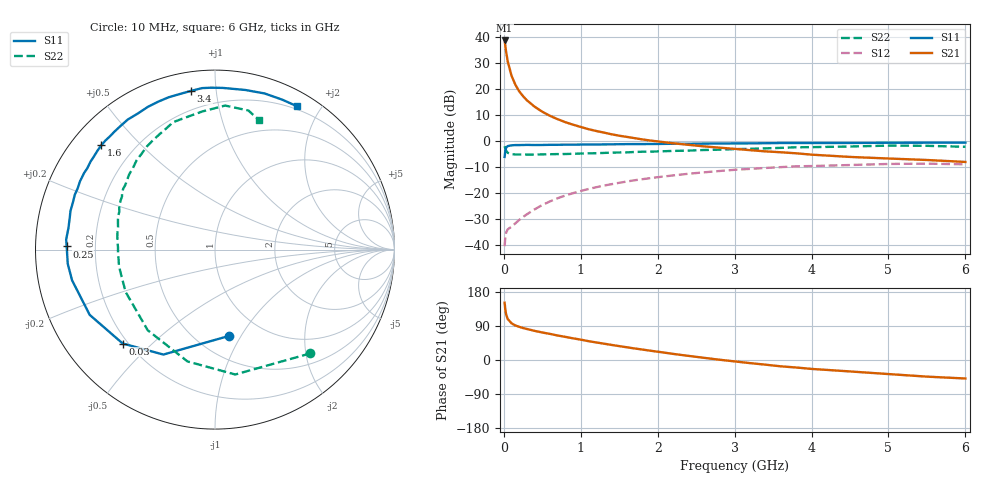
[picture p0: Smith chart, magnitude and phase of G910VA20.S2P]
! SIEMENS Small Signal Semiconductors
! BFG235
! Si NPN RF Bipolar Junction Transistor in SOT223
! VCE = 10 V  IC = 200 mA
! Common Emitter S-Parameters:  July  1994
# GHz  S  MA  R  50
!  f  S11  S21  S12  S22
! GHz  MAG  ANG  MAG  ANG  MAG  ANG  MAG  ANG
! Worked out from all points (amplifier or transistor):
!   40 points, 10 MHz to 6 GHz, reference 50 ohm
!   highest |S21| = 38.6 dB at 10 MHz (marker M1)
!   |S21| within 3 dB of that: start of sweep to 23.6 MHz
!   unconditionally stable (mu >= 1): 410.2 MHz to 1.514 GHz
!   at 200 MHz: K = 0.81, MSG = 24.8 dB, |S12| = -30.5 dB
!   at 1.5 GHz: K = 1.00, MAG = 8.8 dB, |S12| = -16.2 dB
!   at 6 GHz: K = 0.89, MSG = 0.5 dB, |S12| = -9.1 dB
!   S11 on the Smith chart (normalised r, x): 10 MHz: 0.71, -0.89; 30 MHz: 0.18, -0.41; 250 MHz: 0.09, +0.01; 1.6 GHz: 0.09, +0.39; 3.4 GHz: 0.10, +0.86; 6 GHz: 0.16, +1.72
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0.01  0.487 -80.5  85.33 151.2  0.0093 60.6  0.7854 -47.4
0.02  0.6517 -116.2  66.18 132.0  0.0143 47.0  0.705 -80.8
0.03  0.7336 -134.5  51.35 120.4  0.017 40.0  0.6417 -103.8
0.05  0.7872 -152.5  33.88 108.2  0.0196 32.9  0.585 -129.9
0.1  0.8145 -167.9  17.82 96.8  0.0221 36.5  0.5511 -154.6
0.15  0.8242 -174.5  11.94 91.1  0.0256 43.4  0.5415 -164.8
0.2  0.824 -178.1  8.938 87.5  0.0298 48.8  0.5429 -170.3
0.25  0.8266 178.8  7.2 84.3  0.034 52.1  0.5399 -174.0
0.3  0.8311 176.1  6.01 81.8  0.0383 55.4  0.5408 -177.1
0.4  0.8253 171.6  4.522 76.9  0.0476 58.4  0.5405 178.7
0.5  0.828 168.0  3.61 72.6  0.0577 59.8  0.5451 175.4
0.6  0.8335 165.0  3.012 68.9  0.0678 60.2  0.5491 172.3
0.7  0.8345 161.3  2.596 64.6  0.0781 60.2  0.5525 169.5
0.9  0.8377 155.9  2.033 57.2  0.0977 58.1  0.5597 165.0
1.1  0.845 149.6  1.668 49.7  0.1174 55.8  0.5711 160.3
1.6  0.8597 137.4  1.183 33.6  0.1638 47.5  0.5965 150.3
2.2  0.8724 124.0  0.893 16.1  0.2144 36.7  0.6361 138.7
3.2  0.8887 102.8  0.658 -8.2  0.2868 17.5  0.6984 120.2
3.4  0.8943 98.6  0.623 -12.3  0.2983 13.5  0.7124 115.9
4.5  0.9052 79.3  0.487 -30.2  0.3401 -7.2  0.7726 95.3
5.5  0.9155 65.9  0.425 -43.9  0.3614 -25.6  0.797 76.5
6  0.9202 60.1  0.39 -48.8  0.3508 -32.6  0.763 71.4
